FUNCTION FC 108 : VOID
TITLE =CYCLE OF JOB ROBOT AND FEEDER WITH PRESS
AUTHOR : Esposito
FAMILY : EGAL_srl
NAME : CYCLE_CO
VERSION : 0.1

BEGIN
NETWORK
TITLE =RESERVE

NETWORK
TITLE =CONTROL FORMULATIONS CYCLE JOB ROBOT 1 AND 2 ( CYCLE 1 )
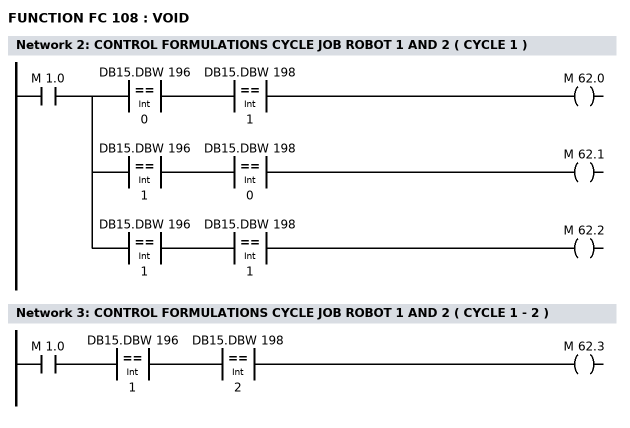
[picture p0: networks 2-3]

      U     M      1.0;
      =     L      0.0;
      U     L      0.0;
      U(    ;
      L     DB15.DBW  196;
      L     0;
      ==I   ;
      )     ;
      U(    ;
      L     DB15.DBW  198;
      L     1;
      ==I   ;
      )     ;
      =     M     62.0;
      U     L      0.0;
      U(    ;
      L     DB15.DBW  196;
      L     1;
      ==I   ;
      )     ;
      U(    ;
      L     DB15.DBW  198;
      L     0;
      ==I   ;
      )     ;
      =     M     62.1;
      U     L      0.0;
      U(    ;
      L     DB15.DBW  196;
      L     1;
      ==I   ;
      )     ;
      U(    ;
      L     DB15.DBW  198;
      L     1;
      ==I   ;
      )     ;
      =     M     62.2;
NETWORK
TITLE =CONTROL FORMULATIONS CYCLE JOB ROBOT 1 AND 2 ( CYCLE 1 - 2 )

      U     M      1.0;
      U(    ;
      L     DB15.DBW  196;
      L     1;
      ==I   ;
      )     ;
      U(    ;
      L     DB15.DBW  198;
      L     2;
      ==I   ;
      )     ;
      =     M     62.3;
END_FUNCTION

